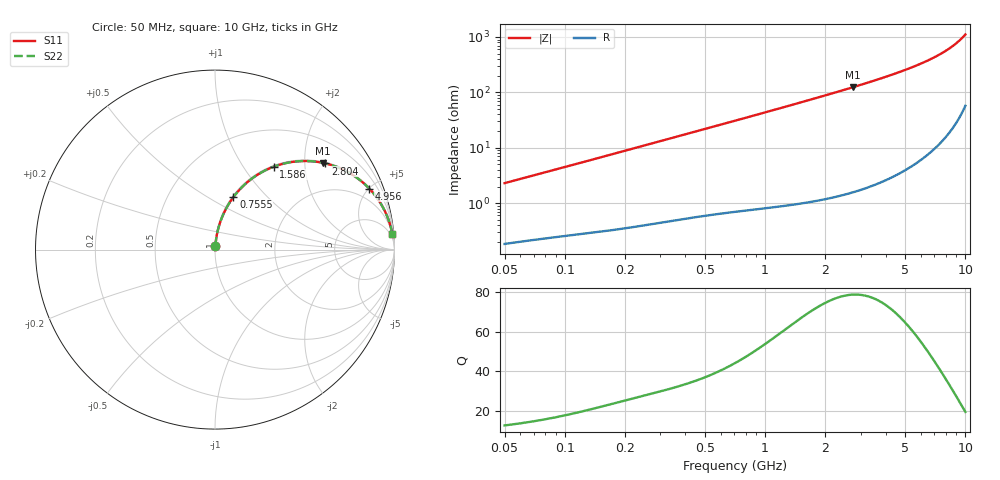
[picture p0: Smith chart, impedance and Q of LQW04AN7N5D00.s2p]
!Murata Part Number: LQW04AN7N5D00
!These Parameters are Measured in Series Mode Connection
!  o--[Z]--o
!Port1  Port2
!  o-------o
!Freq. Start=50[MHz] Stop=10[GHz], 401[Steps]
# Hz S RI R 50
!Freq.(Hz)	S 11(Real)	S 11(Imag)	S 21(Real)	S 21(Imag)	S 12(Real)	S 12(Imag)	S 22(Real)	S 22(Imag)
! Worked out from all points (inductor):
!   401 points, 50 MHz to 10 GHz, reference 50 ohm
!   read as one part in series: L = 7.24 nH near 51.34 MHz
!   highest Q = 78.8 at 2.731 GHz (marker M1), where L = 7.18 nH
!   S11 on the Smith chart (normalised r, x): 50 MHz: 1.00, +0.05; 755.5 MHz: 1.01, +0.66; 1.586 GHz: 1.02, +1.39; 2.804 GHz: 1.03, +2.54; 4.956 GHz: 1.08, +5.02; 10 GHz: 2, +22
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5e7  0.00236 0.0228  0.9976 -0.0228  0.9976 -0.0228  0.00236 0.0228
1.214486e8  0.00568 0.0538  0.9943 -0.0538  0.9943 -0.0538  0.00568 0.0538
1.956524e8  0.0108 0.0854  0.9892 -0.0854  0.9892 -0.0854  0.0108 0.0854
2.949953e8  0.0207 0.1265  0.9793 -0.1265  0.9793 -0.1265  0.0207 0.1265
4.81571e8  0.0474 0.1991  0.9526 -0.1991  0.9526 -0.1991  0.0474 0.1991
7.071068e8  0.0917 0.2775  0.9083 -0.2775  0.9083 -0.2775  0.0917 0.2775
7.555233e8  0.1026 0.2927  0.8974 -0.2927  0.8974 -0.2927  0.1026 0.2927
9.215873e8  0.1432 0.3406  0.8568 -0.3406  0.8568 -0.3406  0.1432 0.3406
1.10936e9  0.1933 0.3862  0.8067 -0.3862  0.8067 -0.3862  0.1933 0.3862
1.31782e9  0.2517 0.4261  0.7483 -0.4261  0.7483 -0.4261  0.2517 0.4261
1.586325e9  0.3278 0.4622  0.6722 -0.4622  0.6722 -0.4622  0.3278 0.4622
1.717543e9  0.3642 0.4742  0.6358 -0.4742  0.6358 -0.4742  0.3642 0.4742
2.179987e9  0.4834 0.4932  0.5166 -0.4932  0.5166 -0.4932  0.4834 0.4932
2.730534e9  0.6013 0.4833  0.3987 -0.4833  0.3987 -0.4833  0.6013 0.4833
2.803837e9  0.615 0.4803  0.385 -0.4803  0.385 -0.4803  0.615 0.4803
3.375117e9  0.7066 0.4489  0.2934 -0.4489  0.2934 -0.4489  0.7066 0.4489
4.171863e9  0.7981 0.3946  0.2019 -0.3946  0.2019 -0.3946  0.7981 0.3946
4.955797e9  0.8591 0.3403  0.1409 -0.3403  0.1409 -0.3403  0.8591 0.3403
6.207365e9  0.9201 0.2619  0.0799 -0.2619  0.0799 -0.2619  0.9201 0.2619
7.472112e9  0.9553 0.1946  0.0447 -0.1946  0.0447 -0.1946  0.9553 0.1946
8.644138e9  0.9747 0.1415  0.0253 -0.1415  0.0253 -0.1415  0.9747 0.1415
1e10  0.9874 0.0885  0.0126 -0.0885  0.0126 -0.0885  0.9874 0.0885
